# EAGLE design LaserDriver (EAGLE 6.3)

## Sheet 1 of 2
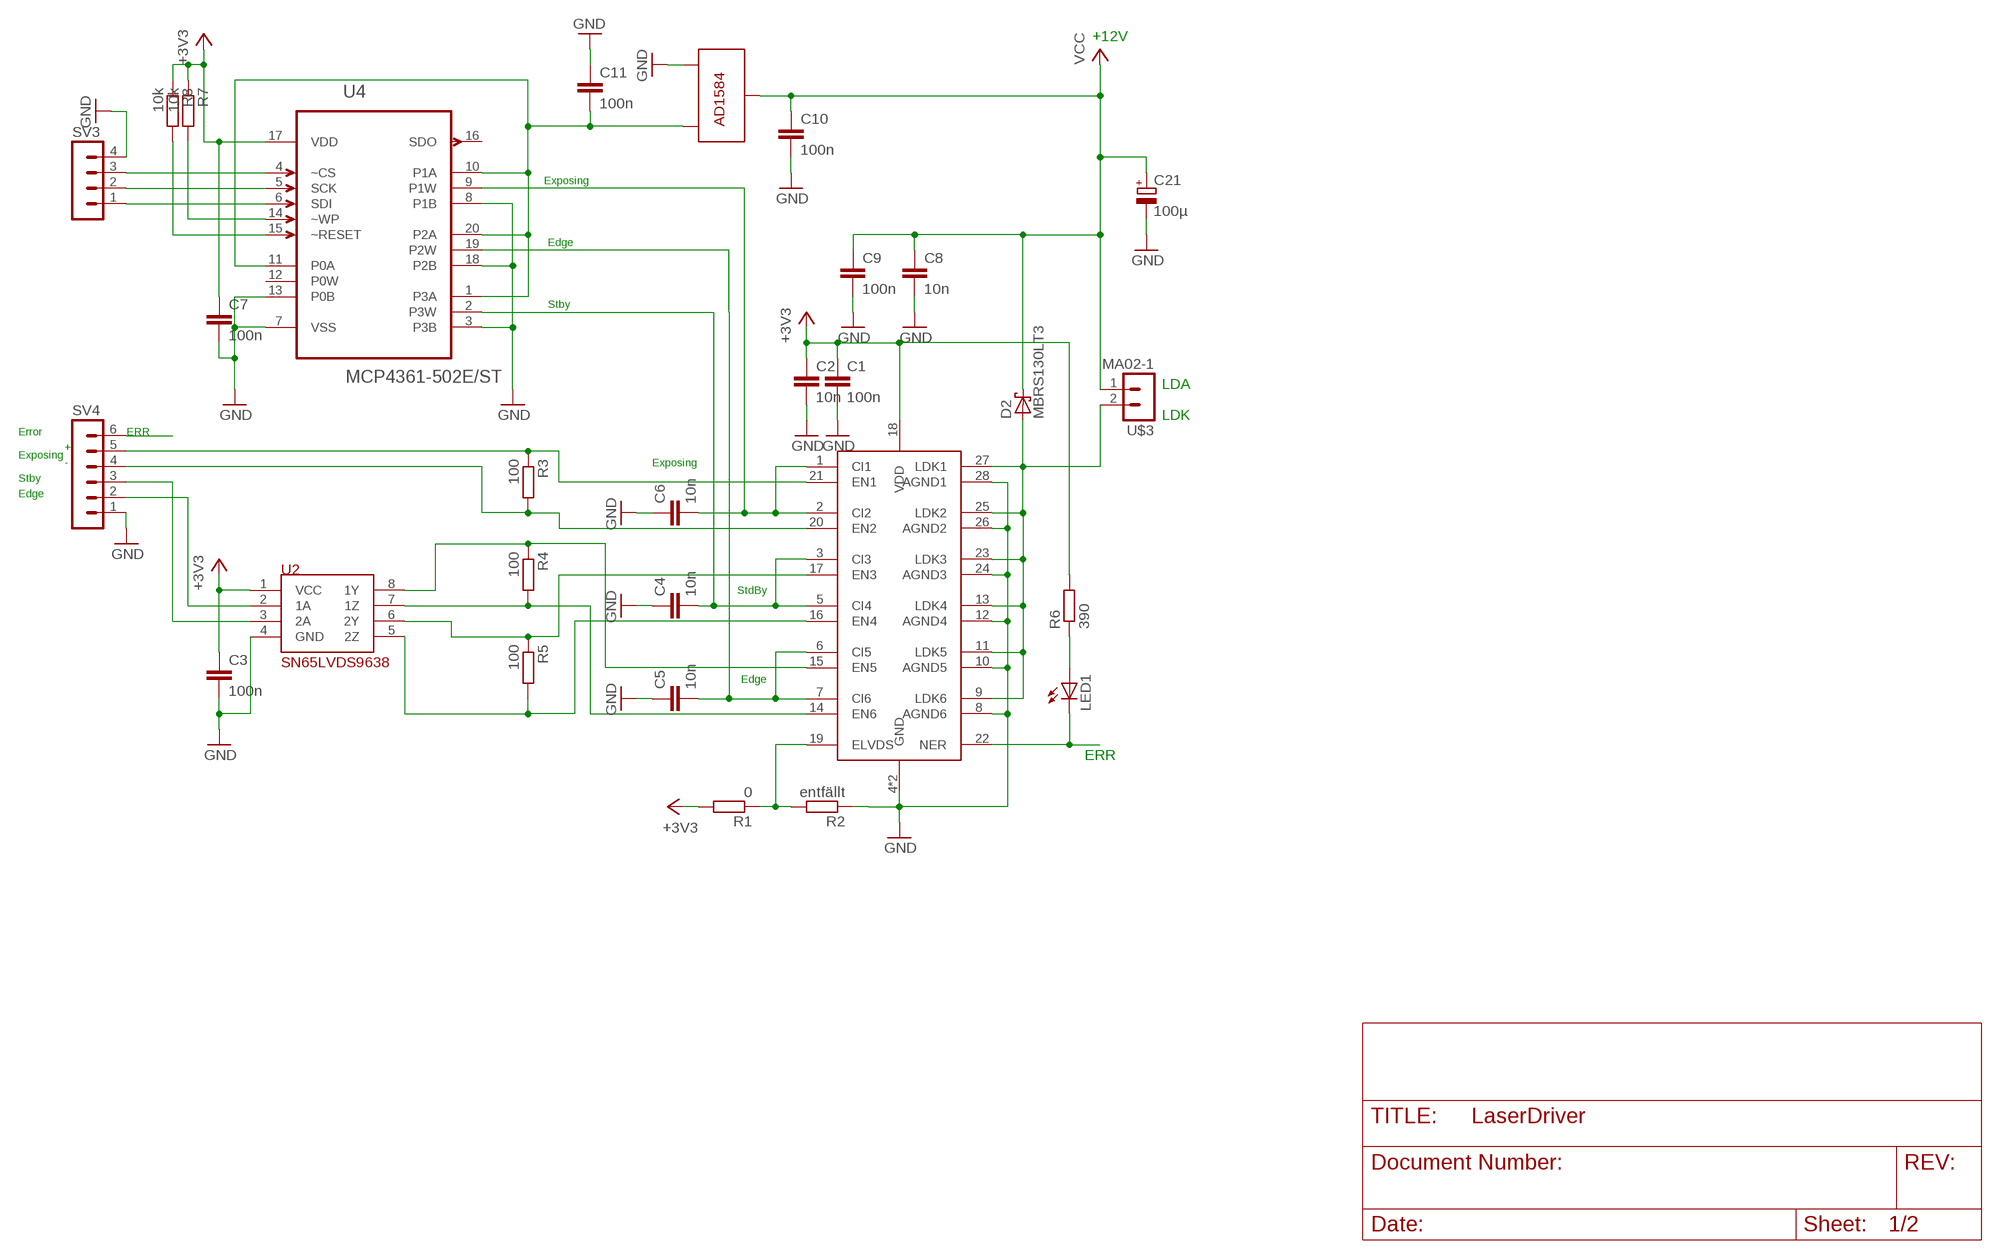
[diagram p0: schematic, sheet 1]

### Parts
C1  100n  C-EUC0805  [C0805]
C2  10n  C-EUC0805  [C0805]
C3  100n  C-EUC0805  [C0805]
C4  10n  C-EUC0805  [C0805]
C5  10n  C-EUC0805  [C0805]
C6  10n  C-EUC0805  [C0805]
C7  100n  C-EUC0805  [C0805]
C8  10n  C-EUC0805  [C0805]
C9  100n  C-EUC0805  [C0805]
C10  100n  C-EUC0805  [C0805]
C11  100n  C-EUC0805  [C0805]
C21  100µ  CPOL-EU153CLV-0505  [153CLV-0505]
D2  MBRS130LT3  [SMB]
LED1  LEDCHIP-LED0805  [CHIP-LED0805]
R1  0  R-EU_M0805  [M0805]
R2  entfällt  R-EU_M0805  [M0805]
R3  100  R-EU_R0805  [R0805]
R4  100  R-EU_R0805  [R0805]
R5  100  R-EU_R0805  [R0805]
R6  390  R-EU_M0805  [M0805]
R7  10k  R-EU_M0805  [M0805]
R8  10k  R-EU_M0805  [M0805]
SV3  MA04-1  [MA04-1]
SV4  MA06-1  [MA06-1]
U1  IC-HG  [QFN28]
U2  SN65LVDS9638  [SOIC8]
U4  MCP4361-502E/ST  [SOP65P640X120-20N]
U6  AD1584B  [SOT-23]
U$3  MA02-1  [MA02-1]

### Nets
+3V3: C1.1 C2.1 C3.1 C7.1 R1.2 R6.2 R7.1 R8.1 U1.18(VDD) U2.1(VCC) U4.17(VDD) ; also sheet 2
ERR: LED1.C SV4.6 U1.22(NER)
GND: C1.2 C2.2 C3.2 C4.1 C5.1 C6.1 C7.2 C8.2 C9.2 C10.2 C11.1 C21.- R2.1 SV3.4 SV4.1 U1.4(GND) U1.8(AGND6) U1.10(AGND5) U1.12(AGND4) U1.24(AGND3) U1.26(AGND2) U1.28(AGND1) U1.GND@1(GND) U2.4(GND) U4.3(P3B) U4.7(VSS) U4.8(P1B) U4.13(P0B) U4.18(P2B) U6.2 ; also sheet 2
N$1: R1.1 R2.2 U1.19(ELVDS)
N$2: D2.A U1.9(LDK6) U1.11(LDK5) U1.13(LDK4) U1.23(LDK3) U1.25(LDK2) U1.27(LDK1) U$3.2
N$3: R3.1 SV4.5 U1.21(EN1)
N$4: R3.2 SV4.4 U1.20(EN2)
N$5: R4.1 U1.15(EN5) U2.8(1Y)
N$6: R4.2 U1.14(EN6) U2.7(1Z)
N$7: R5.1 U1.17(EN3) U2.6(2Y)
N$8: R5.2 U1.16(EN4) U2.5(2Z)
N$9: C11.2 U4.1(P3A) U4.10(P1A) U4.11(P0A) U4.20(P2A) U6.3
N$10: SV3.3 U4.4(~CS)
N$11: SV3.2 U4.5(SCK)
N$12: SV3.1 U4.6(SDI)
N$13: SV4.2 U2.2(1A)
N$14: C5.2 U1.6(CI5) U1.7(CI6) U4.19(P2W)
N$15: C6.2 U1.1(CI1) U1.2(CI2) U4.9(P1W)
N$16: R8.2 U4.15(~RESET)
N$17: LED1.A R6.1
N$19: R7.2 U4.14(~WP)
N$20: C4.2 U1.3(CI3) U1.5(CI4) U4.2(P3W)
N$21: SV4.3 U2.3(2A)
VCC: C8.1 C9.1 C10.1 C21.+ D2.C U6.1 U$3.1 ; also sheet 2
Unconnected: U4.12(P0W) U4.16(SDO)

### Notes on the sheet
- +12V
- Exposing
- Edge
- Stby
- LDA
- LDK
- Error | ERR
- +
- Exposing
- - | Exposing
- Stby
- Edge
- StdBy
- Edge
- ERR

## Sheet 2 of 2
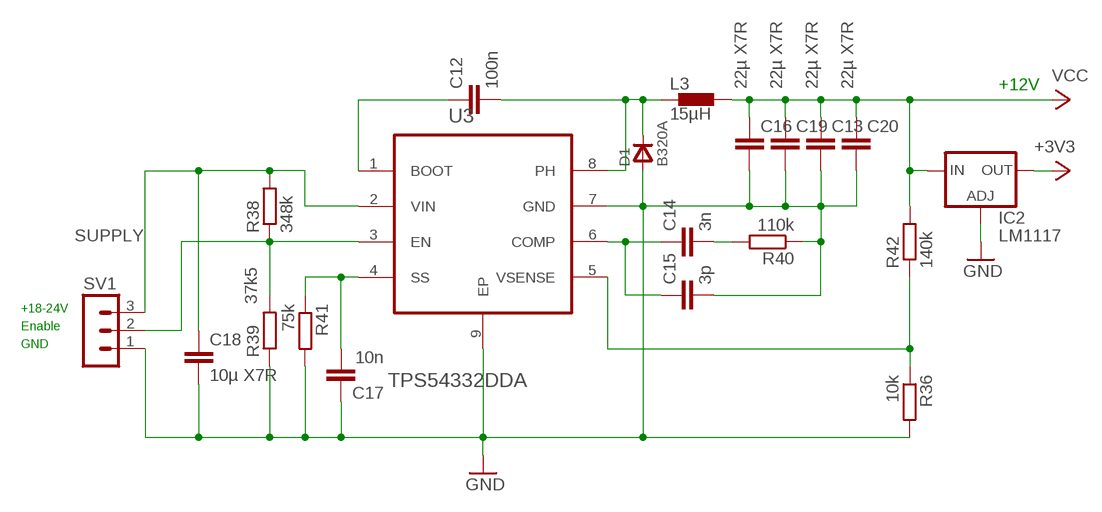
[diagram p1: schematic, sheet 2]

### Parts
C12  100n  C-EUC0805  [C0805]
C13  22µ X7R  C-EUC1210  [C1210]
C14  3n  C-EUC0805  [C0805]
C15  3p  C-EUC0805  [C0805]
C16  22µ X7R  C-EUC1210  [C1210]
C17  10n  C-EUC0805  [C0805]
C18  10µ X7R  C-EUC1210  [C1210]
C19  22µ X7R  C-EUC1210  [C1210]
C20  22µ X7R  C-EUC1210  [C1210]
D1  B320A  DSMA  [DSMA]
IC2  LM1117  LD117AS50TR  [SOT223]
L3  15µH  DR1030  [DR1030]
R36  10k  R-EU_M0805  [M0805]
R38  348k  R-EU_M0805  [M0805]
R39  37k5  R-EU_M0805  [M0805]
R40  110k  R-EU_M0805  [M0805]
R41  75k  R-EU_M0805  [M0805]
R42  140k  R-EU_R0805  [R0805]
SV1  MA03-1  [MA03-1]
U3  TPS54332DDA  [SOIC127P600X170-9N]

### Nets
+3V3: IC2.4(OUT) ; also sheet 1
GND: C13.2 C15.2 C16.2 C17.1 C18.2 C19.2 C20.2 D1.A IC2.1(ADJ) R36.2 R39.1 R40.1 R41.2 SV1.1 U3.7(GND) U3.9(EP) ; also sheet 1
LASER_SUPPLY_EN: R38.1 R39.2 SV1.2 U3.3(EN)
N$26: R36.1 R42.1 U3.5(VSENSE)
N$27: C12.1 U3.1(BOOT)
N$28: C14.1 C15.1 U3.6(COMP)
N$29: C14.2 R40.2
N$30: C17.2 R41.1 U3.4(SS)
N$32: C12.2 D1.C L3.1 U3.8(PH)
SUPPLY: C18.1 R38.2 SV1.3 U3.2(VIN)
VCC: C13.1 C16.1 C19.1 C20.1 IC2.3(IN) L3.2 R42.2 ; also sheet 1

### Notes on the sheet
- +12V
- +18-24V
- Enable
- GND

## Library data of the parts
C1-C20 = rcl:C-EU: CAPACITOR, European symbol
C21 = rcl:CPOL-EU: POLARIZED CAPACITOR, European symbol
D1 = diodes:D: Diode
D2 = diode:MBRS130LT3: Schottky Power Rectifier
IC2 = v-reg:LD117A?*: Low drop fixed and adjustable positive voltage regulators 1 A Source: http://www.st.com/stonline/products/literature/ds/7194/ld1117axx.pdf
L3 = inductors:DR1030: DR1030 Series Low Profile Power Inductors
LED1 = led:LED: LED
R1-R8 R36 R38-R42 = rcl:R-EU_: RESISTOR, European symbol
SV1 = con-lstb:MA03-1: PIN HEADER; OC_FARNELL: unknown; OC_NEWARK: unknown
SV3 = con-lstb:MA04-1: PIN HEADER; OC_FARNELL: unknown; OC_NEWARK: unknown
SV4 = con-lstb:MA06-1: PIN HEADER; OC_FARNELL: unknown; OC_NEWARK: unknown
U1 = ic-haus:IC-HG
U2 = ic-haus:SN65LVDS9638
U3 = tps54332:TPS54332DDA: 3.5A, 28V, 1MHz, STEP DOWN SWIFT DC/DC CONVERTER WITH Eco-mode; MPN: TPS54332DDA; OC_FARNELL: 1710821; OC_NEWARK: 50P9395; PACKAGE: SOIC-8; SUPPLIER: Texas Instruments
U4 = Microchip_By_element14_Batch_1:MCP4361-502E/ST: Digital POT; MPN: MCP4361-502E/ST; OC_FARNELL: 1840706; OC_NEWARK: 53R0044; PACKAGE: SOP-20; SUPPLIER: Microchip
U6 = analog-devices:AD1584B
U$3 = con-lstb:MA02-1

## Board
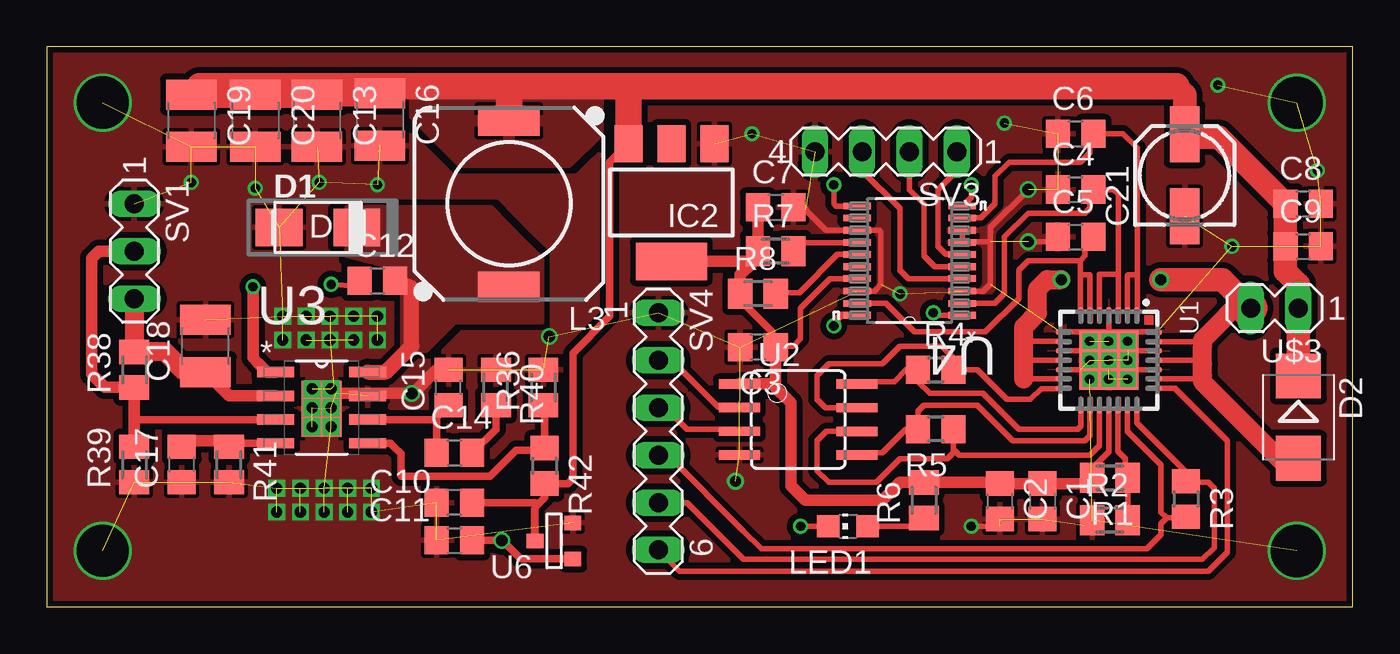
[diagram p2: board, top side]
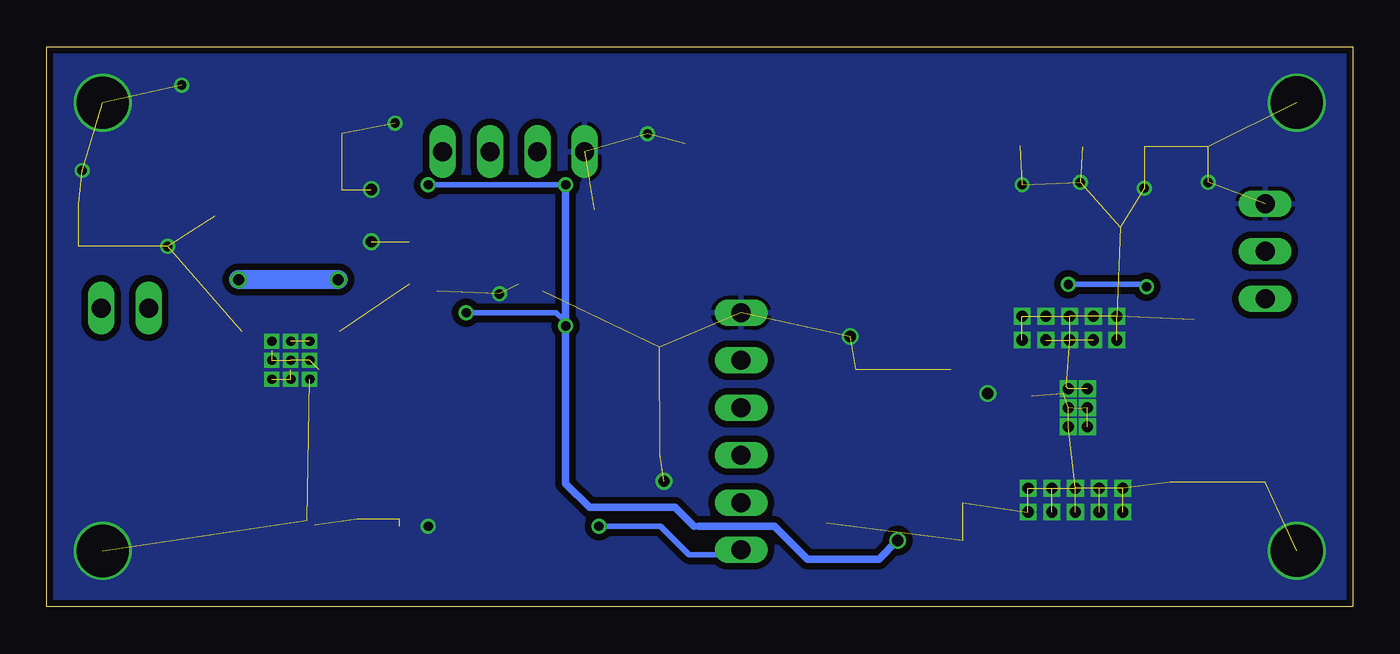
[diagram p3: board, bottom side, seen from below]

Size 69.97 x 30 mm. Coordinates in mm from the lower left corner, seen from the top.
Outline: 0,0 69.97,0 69.97,30 0,30 0,0
Copper layers (1*16): Top 0.035mm / dielectric 1.5mm / Bottom 0.035mm
Design rules "PCB-POOL Standard": minimum track width 0.15mm, minimum drill 0.3mm, track to track 0.15mm, track to pad 0.15mm, pad to pad 0.15mm, via to via 0.15mm, smd to smd 0.15mm, copper to edge 0.3mm, drill to drill 0.2mm, minimum pad ring 0.2mm, minimum via ring 0.15mm, stop-mask expansion 0.075mm, vias tented up to drill 0mil, thermal gap 0.2mm

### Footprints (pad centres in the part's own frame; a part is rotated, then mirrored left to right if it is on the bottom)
C0805 = smd 1.3 x 1.5: 1 -0.95,0; 2 0.95,0
C1210 = smd 1.6 x 2.7: 1 -1.4,0; 2 1.4,0
153CLV-0505 = smd 3 x 1.6: + 2.2,0; - -2.2,0
DSMA = smd 2.5 x 2: A -2.083,0; C 2.083,0
SMB = smd 2.4 x 2.4: A 2.2,0; C -2.2,0
SOT223 = smd 1.5 x 2: 1 -2.3,-3.15; 2 0,-3.15; 3 2.3,-3.15 | smd 3.8 x 2: 4 0,3.15
DR1030 = smd 3.3 x 1.6: 1 0,4.45; 2 0,-4.45
CHIP-LED0805 = smd 1.2 x 1.2: A 0,-1.05; C 0,1.05
M0805 = smd 1.3 x 1.6: 1 -0.95,0; 2 0.95,0
R0805 = smd 1.3 x 1.5: 1 -0.95,0; 2 0.95,0
MA03-1 = drill 1.016 long: 1 -2.54,0; 2 0,0; 3 2.54,0
MA04-1 = drill 1.016 long: 1 -3.81,0; 2 -1.27,0; 3 1.27,0; 4 3.81,0
MA06-1 = drill 1.016 long: 1 -6.35,0; 2 -3.81,0; 3 -1.27,0; 4 1.27,0; 5 3.81,0; 6 6.35,0
QFN28 = smd 0.9 x 0.3: 1 -2.4,1.5; 2 -2.4,1; 3 -2.4,0.5; 4 -2.4,0; 5 -2.4,-0.5; 6 -2.4,-1; 7 -2.4,-1.5; 15 2.4,-1.5; 16 2.4,-1; 17 2.4,-0.5; 18 2.4,0; 19 2.4,0.5; 20 2.4,1; 21 2.4,1.5 | smd 0.3 x 0.9: 8 -1.5,-2.4; 9 -1,-2.4; 10 -0.5,-2.4; 11 0,-2.4; 12 0.5,-2.4; 13 1,-2.4; 14 1.5,-2.4; 22 1.5,2.4; 23 1,2.4; 24 0.5,2.4; 25 0,2.4; 26 -0.5,2.4; 27 -1,2.4; 28 -1.5,2.4 | smd 3.15 x 3.15: GND@1 0,0
SOIC8 = smd 0.5 x 2.2: 1 -1.905,-3.154; 2 -0.645,-3.154; 3 0.625,-3.154; 4 1.895,-3.154; 5 1.905,3.154; 6 0.635,3.154; 7 -0.635,3.154; 8 -1.905,3.154
SOIC127P600X170-9N = smd 1.981 x 0.559: 1 -2.464,1.905; 2 -2.464,0.635; 3 -2.464,-0.635; 4 -2.464,-1.905; 5 2.464,-1.905; 6 2.464,-0.635; 7 2.464,0.635; 8 2.464,1.905 | smd 2.134 x 2.997: 9 0,-0.051
SOP65P640X120-20N = smd 1.473 x 0.356: 1 -2.819,2.921; 2 -2.819,2.286; 3 -2.819,1.626; 4 -2.819,0.965; 5 -2.819,0.33; 6 -2.819,-0.33; 7 -2.819,-0.965; 8 -2.819,-1.626; 9 -2.819,-2.286; 10 -2.819,-2.921; 11 2.819,-2.921; 12 2.819,-2.286; 13 2.819,-1.626; 14 2.819,-0.965; 15 2.819,-0.33; 16 2.819,0.33; 17 2.819,0.965; 18 2.819,1.626; 19 2.819,2.286; 20 2.819,2.921
SOT-23 = smd 0.787 x 0.889: 1 0.025,-1.016; 2 -0.94,1.016; 3 0.991,1.016
MA02-1 = drill 1.016 long: 1 -2.54,0; 2 0,0

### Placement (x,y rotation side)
C1  53.34,5.65 270 top
C2  51.05,5.65 270 top
C3  38.1,13.91 180 top
C4  55.12,22.35 0 top
C5  55.12,19.81 0 top
C6  55.12,25.34 0 top
C7  39.05,21.4 0 top
C8  67.31,21.59 0 top
C9  67.31,19.3 0 top
C10  21.84,5.59 180 top
C11  21.84,3.56 0 top
C12  17.72,17.46 0 top
C13  14.48,26.04 270 top
C14  21.84,8.25 0 top
C15  21.53,11.75 90 top
C16  17.84,26.1 270 top
C17  7.24,7.62 90 top
C18  8.51,13.97 90 top
C19  7.75,26.04 270 top
C20  11.18,26.04 270 top
C21  60.96,23.11 90 top
D1  14.54,20.32 0 top
D2  67.06,10.16 270 top
IC2  33.46,21.65 180 top
L3  24.77,21.59 180 top
LED1  42.93,4.32 90 top
R1  56.96,6.92 180 top
R2  56.96,4.64 0 top
R3  61.02,5.78 270 top
R4  47.63,12.7 0 top
R5  47.63,9.52 180 top
R6  46.99,5.71 90 top
R7  39.05,19.05 0 top
R8  38.1,16.76 0 top
R36  26.61,11.75 90 top
R38  4.7,12.7 90 top
R39  4.7,7.62 90 top
R40  24.07,11.75 270 top
R41  9.78,7.62 270 top
R42  26.67,7.56 270 top
SV1  4.7,19.05 270 top
SV3  44.96,24.38 180 top
SV4  32.77,9.4 270 top
U1  56.9,13.21 270 top
U2  40.26,10.03 270 top
U3  14.73,10.67 0 top
U4  46.23,18.54 180 top
U6  27.18,3.56 270 top
U$3  64.52,16 180 top

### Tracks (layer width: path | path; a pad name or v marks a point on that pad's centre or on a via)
+3V3
  Top 0.305: U1.18 56.9,8.64 56.9,8.32 55.88,7.3 55.88,7.05 R1.2 55.82,6.92 55.88,6.99 | 55.88,7.11 55.88,6.99 | 55.88,6.99 55.88,6.79 | 39.37,13.9 C3.1 | 32.92,19.05 IC2.4 | U4.17 41.96,17.58 40.39,16 40.39,14.73 40.39,14.35 40.01,13.97 39.11,13.97 C3.1 | R8.1 37.15,16.44 | 38.86,14.73 38.86,14.41 C3.1 | 50.99,6.35 C2.1 50.99,6.35
  Top 0.406: 50.99,6.35 C2.1 | R8.1 37.15,16.44 38.86,14.73
  Top 0.61: 39.88,7.43 | R1.2 55.37,6.6 C1.1 C2.1 50.99,6.67 R6.2 45.72,6.67 44.77,5.72 40.64,5.72 40.01,6.35 39.88,6.48 39.88,7.43 | C7.1 R7.1 | R7.1 38.1,18.74 37.78,18.42 | 37.78,18.42 37.15,17.78 R8.1 | 38.01,19.14 R7.1 | C3.1 39.05,12.07 39.05,11.75 | 39.05,11.75 39.69,11.11 39.88,10.92 39.88,7.43 | U2.1 38.86,11.94 39.05,11.75 | IC2.4 37.69,18.5 37.78,18.42
ERR  (via drill 0.5)
  Top 0.305: U1.22 60.46,11.71 60.46,11.67 61.98,10.16 63.25,8.89 63.25,2.92 62.23,1.91 33.91,1.91 SV4.6 | LED1.C v40.39,4.32
  Bottom 0.305: v40.39,4.32 37.08,4.32 35.56,2.79 33.02,2.79 SV4.6
GND  (via drill 0.5, 0.6, 2.8)  (84 unrouted)
  Top 0.305: U1.4 56.9,14.73 | 56.9,14.73 v56.9,14.22 | 56.9,12.71 U1.GND@1 56.9,13.72 54.3,13.72 U1.10 | 56.9,12.71 56.9,12.7 | U1.8 54.3,14.73 56.9,14.73 | 56.9,12.71 U1.24 | U1.26 59.5,13.72 57.91,13.72 v57.91,14.22 | U1.28 59.5,14.73 56.9,14.73 | U1.12 55.36,12.71 v55.88,12.19 | U4.18 44.35,16.92 44.45,17.02 44.7,17.27 44.7,20.07 44.6,20.17 U4.13 41.75,20.17 40.64,21.27 | U4.8 U4.7 49.1,19.56 50.29,19.56 50.55,19.56 | U4.3 50.19,16.92 50.55,17.27 50.55,19.56 | v52.58,19.56 53.66,19.56 C5.1 | v49.53,4.32 51.05,4.32 | 50.55,19.56 50.55,20.32 v52.58,22.35 | 55.63,4.38 R2.1
  Top 0.406: 15.37,11.81 15.49,11.43 | v56.9,14.22 56.9,13.72 | 56.9,12.7 56.9,12.71 | 40.64,21.27 40.13,21.27 C7.2
  Top 0.61: 15.49,11.43 v19.56,11.43 19.62,11.43 20.89,12.7 C15.2
  other vias: 12.32,6.35 13.59,6.35 14.86,6.35 16.13,6.35 17.4,6.35 12.32,5.08 13.59,5.08 14.86,5.08 16.13,5.08 17.4,5.08 12.64,15.56 13.91,15.56 15.18,15.56 16.45,15.56 12.64,14.29 13.91,14.29 15.18,14.29 16.45,14.29 17.72,15.56 17.72,14.29 56.9,13.21 55.88,13.21 55.88,14.22 56.9,12.19 57.91,12.19 57.91,13.21 14.22,11.68 15.24,11.68 14.22,10.67 15.24,10.67 14.22,9.65 15.24,9.65 36.89,6.73 45.72,16.76 68.07,23.37 63.5,19.3 37.78,25.34 62.74,27.94 51.31,25.91 7.75,22.73 11.18,22.42 14.61,22.73 17.72,22.61 26.92,14.48 66.97,3 3,3 3,27 66.97,27
  pour Bottom (isolate 0.35, rank 2): 0.32,29.85 0.25,0.25 69.85,0.25 69.85,29.85
  pour Top (isolate 0.32, rank 6): 0.32,29.85 0.25,0.25 69.85,0.25 69.85,29.85
  pour Top (no thermals): 11.94,16.26 11.94,13.72 13.21,13.72 13.97,13.21 13.97,8.64 13.21,7.87 11.94,7.87 11.94,4.57 17.78,4.57 17.78,7.87 16.51,7.87 15.49,8.38 15.49,12.95 16.76,13.72 17.78,13.72 18.29,14.22 18.29,16 16.76,16 16.76,16.26
LASER_SUPPLY_EN
  Top 0.406: R38.1 4.7,10.16 4.83,10.03 U3.3
  Top 0.61: R39.2 4.7,10.16 R38.1 3.11,11.75 2.41,12.45 2.41,18.67 2.79,19.05 SV1.2
N$1
  Top 0.305: 58.1,7.12 R1.1 | R1.1 R2.2 | U1.19 57.4,8.33 57.79,7.94 57.79,7.05 R1.1
N$2  (via drill 0.6)
  Top 0.305: 54.3,12.19 U1.13 52.34,12.21 52.32,12.19 | U1.9 54.3,14.22 52.32,14.22 | U1.11 52.32,13.21 | U1.27 61.68,14.21 61.91,13.97 | U1.25 61.72,13.21 61.91,13.02 | U1.23 61.74,12.21 61.91,12.38
  Top 0.813: 61.91,12.07 61.91,12.38 | 61.91,13.97 61.91,14.29 | 63.5,15.88 64.39,15.88
  Top 1.016: 52.32,12.19 52.32,13.21 52.32,14.22 52.32,14.99 53.09,15.75 53.09,17.02 53.59,17.53 v54.36,17.53 | 66.72,7.62 66.36,7.62 61.91,12.07 | 61.91,12.38 61.91,13.02 61.91,13.97 | 61.91,14.29 62.87,15.24 63.5,15.88
  Top 1.27: 66.72,7.62 D2.A | v59.69,17.53 62.99,17.53 U$3.2
  Top 1.778: 64.39,15.88 U$3.2
  Bottom 1.016: v54.36,17.53 v59.69,17.53
N$3
  Top 0.305: 34.29,5.59 SV4.5 34.29,5.59 | 34.29,5.59 36.58,3.3 37.24,2.64 37.34,2.54 61.91,2.54 62.55,3.18 62.55,6.35 62.23,6.67 61.08,6.67 R3.1 60.96,6.79 60.96,7.3 58.4,9.87 U1.21
N$4
  Top 0.305: SV4.4 33.27,8.13 37.34,4.06 38.29,3.11 58.93,3.11 59.69,3.87 59.69,4.45 60.01,4.76 | U1.20 57.9,9.41 59.37,7.94 59.69,7.62 59.69,5.08 60.01,4.76 | 60.01,4.76 60.96,4.76 R3.2
N$5
  Top 0.254: 46.67,12.07 46.67,13.02 R4.1
  Top 0.305: U1.15 55.4,9.68 55.25,9.53 52.07,9.53 50.17,11.43 47.31,11.43 46.67,12.07 | 43.54,12.07 U2.8 43.54,12.07 | R4.1 46.04,12.7 45.4,12.07 43.54,12.07
N$6
  Top 0.254: 48.89,12.7 R4.2
  Top 0.305: U1.14 54.27,11.68 53.28,11.68 52.71,11.11 51.44,11.11 49.85,12.7 48.89,12.7 | R4.2 48.58,13.34 47.94,13.97 45.72,13.97 44.77,13.02 41.91,13.02 41.28,12.38 41.28,11.11 41.59,10.8 41.72,10.67 U2.7
N$7
  Top 0.254: R5.1 48.58,8.57 48.58,8.45
  Top 0.305: U1.17 56.39,10.6 56.39,8.64 55.88,8.13 48.9,8.13 48.58,8.45 | R5.1 48.58,8.57 48.58,8.25 48.26,7.94 46.36,7.94 45.72,7.94 44.45,6.67 41.91,6.67 41.28,7.3 41.28,8.89 41.59,9.21 41.78,9.4 U2.6
N$8
  Top 0.254: R5.2
  Top 0.305: U1.16 55.9,9.16 55.63,8.89 51.75,8.89 49.85,10.8 46.99,10.8 46.67,10.48 R5.2 | R5.2 46.04,9.53 44.77,8.26 43.54,8.26 U2.5
N$9  (via drill 0.5, 0.6)
  Top 0.305: U4.11 42.8,21.46 42.29,21.46 42.16,21.59 v42.16,22.61 | U4.1 47.63,15.62 v47.5,15.75 | v49.53,22.61 49.53,21.95 U4.10
  Top 0.406: C11.2 23.88,3.56 v24.38,3.56 25.37,2.57 U6.3 | U4.20 42.8,15.62 42.55,15.62 42.16,15.24 v42.16,15.05
  Bottom 0.305: v42.16,22.61 v49.53,22.61 | 35.05,4.32 35.31,4.32 | v47.5,15.75 42.67,15.75 42.29,15.37 42.29,15.62 42.16,15.75
  Bottom 0.406: 35.31,4.32 36.32,5.33 40.89,5.33 42.16,6.6 v42.16,15.05 42.16,15.75 v42.16,22.61 | 35.05,4.32 30.99,4.32 29.21,2.54 25.4,2.54 v24.38,3.56
N$10
  Top 0.305: U4.4 46.18,17.58 45.72,18.03 45.72,21.34 43.69,23.37 SV3.3
N$11
  Top 0.305: SV3.2 46.23,22.35 46.99,21.59 46.99,18.8 47.5,18.29 47.57,18.21 U4.5
N$12
  Top 0.305: U4.6 48.18,18.87 47.75,19.3 47.75,22.35 48.77,23.37 SV3.1
N$13
  Top 0.305: U2.2 36,10.68 33.34,13.34 32.89,13.34 SV4.2
N$14
  Top 0.305: U4.19 44.96,16.26 46.48,14.73 49.02,14.73 50.29,14.73 52.07,16.51 52.07,18.03 52.58,18.54 55.37,18.54 | 55.37,18.54 55.63,18.8 55.63,19.62 C5.2 | 55.37,18.54 55.37,17.78 | 55.37,17.78 55.37,15.83 U1.7 | U1.6 55.9,17.13 55.88,17.78 55.37,17.78
N$15
  Top 0.305: U1.1 58.4,15.77 58.42,15.75 58.42,17.78 | 58.42,17.78 58.42,17.34 58.42,17.78 | U4.9 49.78,20.83 50.04,20.83 50.8,21.59 50.8,23.05 51.56,23.81 52.32,23.81 53.34,23.81 55.37,23.81 55.88,24.32 55.88,25.59 C6.2 57.66,25.34 58.42,24.57 58.42,17.78 | U1.2 57.9,17.73 57.94,17.78 58.42,17.78
N$16
  Top 0.305: U4.15 42.37,18.87 40.32,16.83 39.11,16.83
  Top 0.406: 39.11,16.83 R8.2
N$17
  Top 0.305: LED1.A 46.86,4.32 R6.1
N$18
  Top 0.254: 54.3,10.83 54.3,10.61 54.29,10.61 54.54,10.61
N$19
  Top 0.305: U4.14 40.46,19.51
  Top 0.406: 40.46,19.51 R7.2
N$20
  Top 0.305: U1.5 56.4,17.01 56.39,17.81 57.4,17.81 | 57.4,17.81 57.4,15.82 U1.3 | 57.4,17.81 57.4,18.03 57.4,22.1 57.15,22.35 C4.2 55.88,22.29 55.88,21.34 55.63,21.08 53.09,21.08 52.58,21.08 51.31,19.81 51.31,19.3 51.31,16.76 50.8,16.26 U4.2
N$21
  Top 0.305: SV4.3 33.15,10.67 34.29,9.53 36.99,9.53 U2.3
N$22
  Top 0.254: 59.24,10.61 59.5,10.61 59.5,10.8 59.5,10.83
N$23
  Top 0.254: 54.3,15.49 54.3,15.81 54.59,15.81
N$26
  Top 0.305: 26.67,10.73 R36.1
  Top 0.406: R36.1 26.67,10.73 R42.1 26.55,8.38 25.15,8.38 23.75,6.99 18.99,6.99 18.99,8.19 18.54,8.64 18.42,8.76 U3.5
N$27  (via drill 0.5)
  Top 0.305: C12.1 16.89,17.15 v15.24,17.27
  Top 0.61: 11.68,12.7 11.3,13.08 | 11.3,13.08 11.05,13.34 v11.05,17.15 | U3.1 11.81,12.57 11.3,13.08
  Bottom 0.305: v15.24,17.27 11.18,17.27 v11.05,17.15
N$28
  Top 0.406: C15.1 20.89,10.16 20.89,9.91 | C14.1 20.89,9.91 | U3.6 20.77,10.03 20.89,9.91
N$29
  Top 0.406: C14.2 24.07,9.53 R40.2
N$30
  Top 0.406: 10.1,8.89 R41.1 9.97,8.76 U3.4
  Top 0.61: R41.1 9.46,8.57 9.14,8.89 7.56,8.89 C17.2
N$32
  Top 0.813: U3.8 18.16,12.57 19.56,13.97 19.56,17.08 C12.2
  pour Top (no thermals): 19.3,13.72 20.32,13.72 21.84,15.24 26.54,15.24 26.54,18.67 25.53,19.62 23.81,21.4 16.07,21.4 16.07,18.8 19.05,18.03 19.05,13.97
SUPPLY
  Top 0.61: U3.2 9.91,11.3 9.78,11.3 C18.1 7.43,12.57 | R38.2
  Top 1.016: SV1.3 R38.2 | 7.43,12.57 6.35,13.65 R38.2
VCC
  Top 0.406: 26.16,5.33 U6.1 26.14,3.56 26.14,5.05 26.16,5.59 | 26.16,5.59 26.16,5.33 | 26.16,5.33 26.67,5.84 R42.2 27.94,6.61 28.19,6.86 28.19,13.59 30.16,15.56 30.16,23.8 IC2.3 | 26.16,5.59 C10.1
  Top 1.27: 60.52,27.88 60.96,27.43 C21.+ 61.13,25.15 62.8,25.15 C8.1 C9.1 66.36,17.97 67.06,17.27 U$3.1 D2.C
  Top 1.422: 60.52,27.88 31.12,27.88 | 31.12,27.88 24.77,27.88 | 24.77,27.88 11.43,27.88 | 11.43,27.88 8.19,27.88 C19.1 C20.1 | IC2.3 31.16,27.83 31.12,27.88 | C16.1 14.54,27.5 C13.1 11.87,27.44 11.43,27.88 | L3.2 24.77,27.88
  pour Top: 19.37,28.26 29.53,28.26 29.53,25.4 27.94,23.81 22.23,23.81 19.37,26.67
